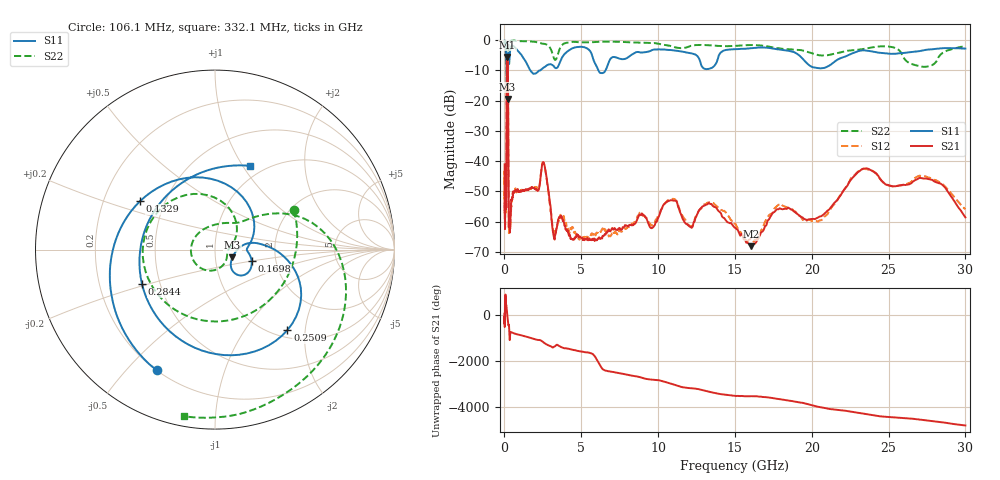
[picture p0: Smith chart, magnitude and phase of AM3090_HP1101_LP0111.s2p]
! Date/Time: Thu, Feb 28, 2019 2:07 PM
! Network Analyzer: Agilent Technologies E8364B Rev: A.07.50.67
! Sweep from 0.010 to 30.000 GHz, 1601 Points, Sweep Type: LOG
! Power Supply: 5.022 V, 0.002 A
# Hz S DB R 50
!freq MagS11 AngS11 MagS21 AngS21 MagS12 AngS12 MagS22 AngS22
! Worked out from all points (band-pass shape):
!   1601 points, 10 MHz to 30 GHz, reference 50 ohm
!   highest |S21| = -5.61 dB at 183.1 MHz (marker M1); lowest = -68.1 dB at 16.05 GHz (marker M2)
!   |S21| within 3 dB of the highest: 151 MHz to 222.6 MHz (71.6 MHz wide, 38.3 % of centre)
!   lowest |S11| = -19.5 dB at 205.4 MHz (marker M3), VSWR 1.24, Z = 60.5 - j5.26 ohm
!   |S11| at or under -10 dB: 144.1 MHz to 229.2 MHz (85.17 MHz wide, 45.6 % of centre); 1.678 GHz to 2.348 GHz (670.8 MHz wide, 33.3 % of centre); 6.11 GHz to 6.583 GHz (473.2 MHz wide, 7.46 % of centre)
!   |S22| runs from -23.0 to -0.2 dB; largest |S21 - S12| = 0.014
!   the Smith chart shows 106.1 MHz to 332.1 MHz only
!   S11 on the Smith chart (normalised r, x): 106.1 MHz: 0.20, -0.61; 132.9 MHz: 0.36, +0.26; 169.8 MHz: 1.50, -0.19; 250.9 MHz: 1.14, -1.61; 284.4 MHz: 0.40, -0.19; 332.1 MHz: 0.86, +1.07
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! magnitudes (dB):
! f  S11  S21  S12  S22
! 10 MHz  -0.3  -41.1  -43.3  -0.6
! 38.04 MHz  -0.4  -59.3  -60.1  -1.3
! 106.1 MHz  -2.5  -54.3  -55.7  -6.2
! 117.9 MHz  -3.6  -52.1  -53.2  -7.8
! 132.9 MHz  -6.1  -28.6  -28.3  -7.9
! 144.7 MHz  -10.3  -12.6  -12.6  -12.3
! 169.8 MHz  -13.4  -5.8  -5.8  -20.4
! 183.1 MHz  -13.1  -5.6  -5.6  -17.6
! 205.4 MHz  -19.5  -6.3  -6.2  -17.6
! 229.3 MHz  -10.0  -11.2  -11.2  -11.8
! 250.9 MHz  -4.4  -33.5  -33.5  -3.0
! 284.4 MHz  -6.9  -61.5  -60.9  -1.0
! 332.1 MHz  -5.9  -59.0  -61.6  -0.5
! 550.5 MHz  -2.0  -50.9  -50.1  -0.3
! 2.084 GHz  -10.9  -49.4  -48.7  -0.7
! 2.584 GHz  -9.0  -41.0  -41.0  -1.3
! 3.236 GHz  -8.9  -65.6  -63.5  -6.2
! 7.926 GHz  -6.1  -61.2  -62.3  -0.8
! 10.86 GHz  -3.4  -52.9  -52.8  -2.0
! 16.05 GHz  -2.7  -68.1  -65.6  -1.7
! 23.36 GHz  -3.4  -42.5  -42.6  -3.0
! 30 GHz  -2.9  -58.6  -55.9  -2.2
